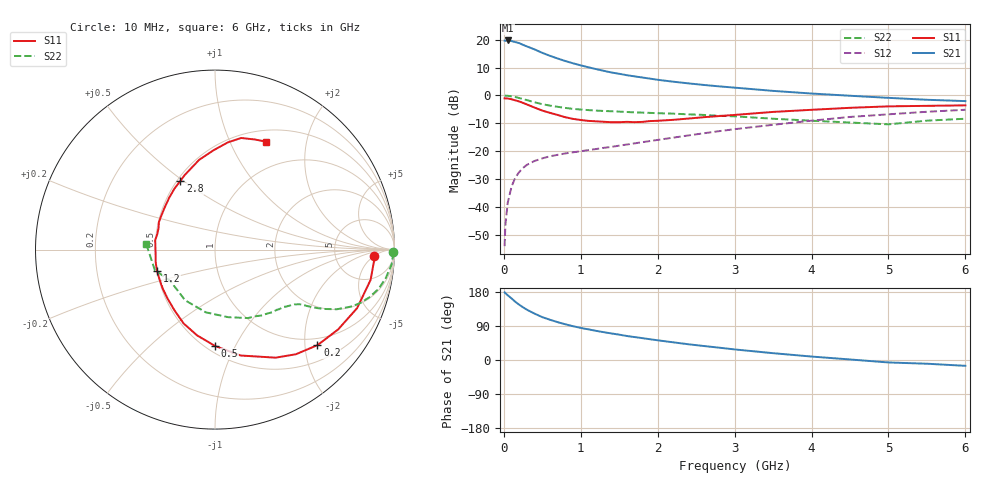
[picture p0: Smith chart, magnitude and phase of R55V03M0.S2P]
! SIEMENS Small Signal Semiconductors
! BFR183
! Si NPN RF Bipolar Junction Transistor in SOT23
! VCE = 5 V  IC = 3 mA
! Common Emitter S-Parameters:  May  1996
# GHz  S  MA  R  50
!  f  S11  S21  S12  S22
! GHz  MAG  ANG  MAG  ANG  MAG  ANG  MAG  ANG
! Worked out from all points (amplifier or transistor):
!   36 points, 10 MHz to 6 GHz, reference 50 ohm
!   highest |S21| = 19.7 dB at 50 MHz (marker M1)
!   |S21| within 3 dB of that: start of sweep to 380.3 MHz
!   unconditionally stable (mu >= 1): 1.27 GHz to 2.766 GHz
!   at 250 MHz: K = 0.30, MSG = 22.0 dB, |S12| = -25.9 dB
!   at 1.4 GHz: K = 1.04, MAG = 12.0 dB, |S12| = -18.4 dB
!   at 6 GHz: K = 0.89, MSG = 1.5 dB, |S12| = -5.1 dB
!   lowest NFmin = 1.10 dB at 450 MHz
!   S11 on the Smith chart (normalised r, x): 10 MHz: 15, -5; 200 MHz: 0.84, -2.28; 500 MHz: 0.55, -0.83; 1.2 GHz: 0.50, -0.13; 2.8 GHz: 0.52, +0.49; 6 GHz: 0.64, +1.38
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0.01  0.889 -2.2  9.597 178.5  0.002 95.1  0.9932 -0.9
0.02  0.8876 -4.5  9.521 176.3  0.0047 85.7  0.9922 -1.9
0.05  0.8833 -11.0  9.675 171.0  0.0119 84.3  0.9875 -4.8
0.1  0.8562 -22.4  9.423 162.5  0.0233 78.2  0.965 -9.4
0.15  0.8175 -33.0  9.04 153.4  0.0341 72.3  0.9372 -13.5
0.2  0.7806 -43.0  8.668 145.9  0.0425 67.8  0.8999 -17.2
0.3  0.6904 -60.7  7.562 132.7  0.0573 60.3  0.8266 -22.5
0.4  0.6071 -76.4  6.685 122.3  0.0673 55.1  0.7556 -26.1
0.5  0.5362 -90.1  5.805 113.1  0.0748 52.1  0.6981 -28.3
0.6  0.4885 -101.7  5.132 106.2  0.0815 50.2  0.6583 -29.7
0.7  0.4477 -112.9  4.596 99.8  0.0866 49.2  0.6268 -30.7
0.8  0.4074 -123.5  4.136 94.2  0.0917 48.6  0.5989 -31.6
0.9  0.381 -133.5  3.771 89.1  0.0961 49.2  0.5756 -32.2
1.1  0.3509 -151.5  3.198 80.8  0.1052 50.2  0.5473 -33.9
1.2  0.3444 -160.0  2.966 76.9  0.11 50.7  0.5362 -34.7
1.6  0.3373 171.0  2.307 63.3  0.1325 53.1  0.5061 -38.9
2.2  0.3661 139.8  1.768 46.7  0.1756 55.4  0.4733 -47.4
2.8  0.4283 116.9  1.456 32.5  0.2297 53.8  0.4328 -59.3
3.5  0.508 100.0  1.209 18.0  0.2986 48.3  0.3833 -79.1
4.5  0.6014 83.2  0.989 1.4  0.4127 37.0  0.3278 -120.5
5.5  0.6524 70.1  0.838 -9.8  0.5108 23.7  0.3542 -161.3
6  0.6655 64.6  0.793 -15.4  0.555 15.0  0.3835 175.6
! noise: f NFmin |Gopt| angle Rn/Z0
0.45  1.1  0.37  35  0.3
0.9  1.15  0.34  85  0.23
1.8  1.9  0.35  160  0.13
